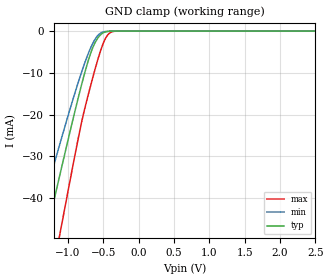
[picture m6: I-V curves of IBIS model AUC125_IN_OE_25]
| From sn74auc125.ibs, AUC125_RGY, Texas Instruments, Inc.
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[Model]   AUC125_IN_OE_25
Model_type  Input
Vinl=0.7
Vinh=1.7
| variable   typ   min   max
C_comp   2.53pF   1.98pF   2.90pF
[Temperature Range]   40   100   -40
| Ambient temperature   25   85   -40
[Voltage range]   2.5   2.3   2.7
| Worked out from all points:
|   GND clamp passes 1 mA (typ) near -0.55 V on its own axis
[GND Clamp]
| AUC125_IN_OE_25
|   Voltage   I(typ)   I(min)   I(max)
-3.6V     -222.6mA   -186.3mA   -267.8mA
-1.485V   -61.97mA   -49.54mA   -81.7mA
-1.435V   -58.22mA   -46.44mA   -77.24mA
-1.3V     -48.12mA   -38.14mA   -65.19mA
-1.115V   -34.46mA   -27.03mA   -48.65mA
-830mV    -14.32mA   -10.98mA   -23.64mA
-720mV    -7.469mA   -5.684mA   -15.68mA
-625mV    -3.065mA   -2.183mA   -9.633mA
-525mV    -682.5uA   -363uA     -4.021mA
-430mV    -73.19uA   -35.01uA   -776.9uA
-325mV    -3.339uA   -2.017uA   -30.74uA
2.5V      328.6pA    415.9pA    485.4pA
